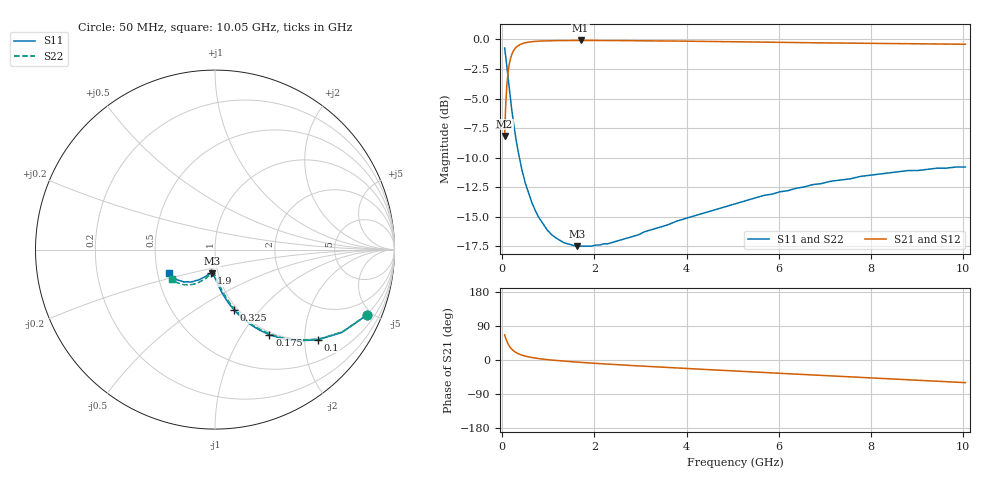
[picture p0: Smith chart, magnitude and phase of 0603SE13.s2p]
! AVX Thin Film Operation		Date: August 2001
! Description: Accu-P® Series, Thin Film, SMD, RF Capacitor
! Part Number: 06035J130FBT
! 50 MHz  -  10.05 GHz
! Serial Measurements
# mhz S db R 50
!	S11		S21		S12		S22
!	dB	Phase	dB	Phase	dB	Phase	dB	Phase
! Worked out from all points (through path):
!   401 points, 50 MHz to 10.05 GHz, reference 50 ohm
!   highest |S21| = -0.08 dB at 1.7 GHz (marker M1); lowest = -8.2 dB at 50 MHz (marker M2)
!   group delay of S21, straight-line fit = 20.1 ps
!   lowest |S11| = -17.5 dB at 1.625 GHz (marker M3), VSWR 1.31, Z = 46.8 - j12.6 ohm
!   |S11| at or under -10 dB: 370.4 MHz to end of sweep
!   |S22| runs from -17.5 to -0.7 dB; largest |S21 - S12| = 0.00011
!   S11 on the Smith chart (normalised r, x): 50 MHz: 0.96, -4.64; 100 MHz: 0.96, -2.32; 175 MHz: 0.96, -1.34; 325 MHz: 0.96, -0.74; 1.9 GHz: 0.93, -0.25; 10.05 GHz: 0.57, -0.17
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50  -0.72 -23.4  -8.18 66.6  -8.18 66.6  -0.72 -23.3
100  -2.35 -41.1  -3.81 49.0  -3.81 49.0  -2.35 -40.8
125  -3.25 -47.7  -2.79 42.4  -2.79 42.4  -3.25 -47.4
175  -4.99 -57.4  -1.66 32.9  -1.66 32.9  -4.99 -56.9
200  -5.79 -61.0  -1.33 29.2  -1.33 29.2  -5.79 -60.4
250  -7.25 -66.6  -0.91 23.7  -0.91 23.7  -7.25 -65.9
325  -9.08 -72.5  -0.58 17.9  -0.58 17.9  -9.08 -71.5
425  -11.02 -77.7  -0.36 12.8  -0.36 12.8  -11.02 -76.5
525  -12.47 -81.2  -0.26 9.4  -0.26 9.4  -12.47 -79.7
675  -14.10 -85.0  -0.18 5.8  -0.18 5.8  -14.10 -83.2
825  -15.27 -87.8  -0.14 3.1  -0.14 3.1  -15.27 -85.6
1125  -16.69 -91.8  -0.10 -0.8  -0.10 -0.8  -16.69 -89.3
1625  -17.50 -96.9  -0.08 -5.7  -0.08 -5.7  -17.50 -93.8
1700  -17.50 -97.6  -0.08 -6.3  -0.08 -6.3  -17.50 -94.5
1725  -17.50 -97.8  -0.08 -6.5  -0.08 -6.5  -17.50 -94.7
1900  -17.50 -99.2  -0.09 -7.9  -0.09 -7.9  -17.50 -96.0
2350  -17.23 -102.7  -0.09 -11.3  -0.09 -11.3  -17.20 -99.2
3400  -15.92 -109.9  -0.12 -18.5  -0.12 -18.5  -15.92 -105.9
5050  -13.92 -121.4  -0.20 -29.1  -0.20 -29.1  -13.82 -116.4
6725  -12.30 -132.0  -0.28 -39.4  -0.28 -39.4  -12.29 -126.0
8400  -11.29 -143.1  -0.36 -49.7  -0.36 -49.7  -11.29 -136.1
10050  -10.80 -152.8  -0.41 -59.8  -0.41 -59.8  -10.72 -145.6
